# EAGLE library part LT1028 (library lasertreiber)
LT1028 Datasheet
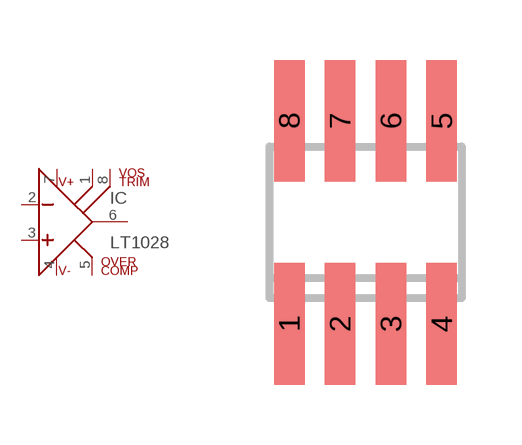
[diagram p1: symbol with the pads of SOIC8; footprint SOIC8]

Designator prefix IC

## LT1028  [SOIC8]
1  VOSTRIM  in
2  IN-  in
3  IN+  in
4  -VS  pwr
5  OVERCOMP  in
6  OUT  out
7  +VS  pwr
8  VOSTRIM  in

## Footprint SOIC8 (pad centres in mm)
Small Outline IC
smd 0.762 x 3.048: 1 -1.905,-2.54; 2 -0.635,-2.54; 3 0.635,-2.54; 4 1.905,-2.54; 5 1.905,2.54; 6 0.635,2.54; 7 -0.635,2.54; 8 -1.905,2.54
